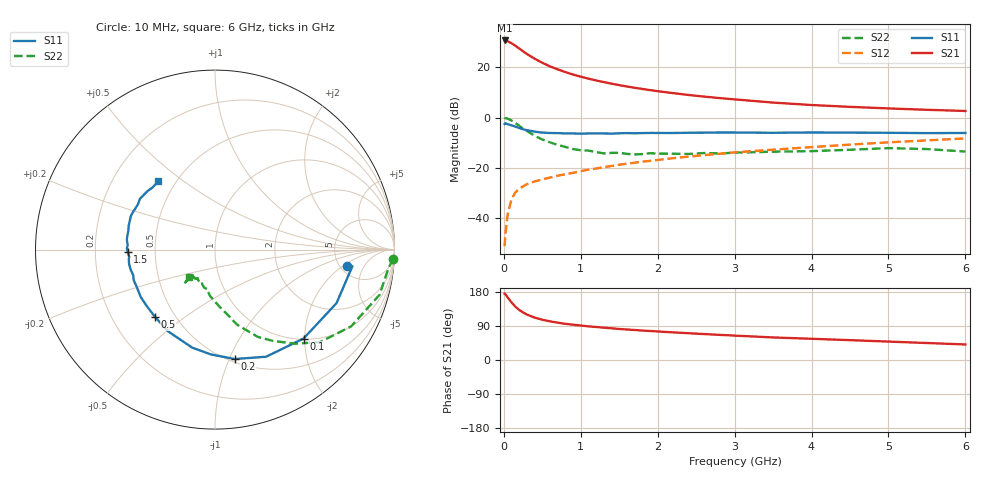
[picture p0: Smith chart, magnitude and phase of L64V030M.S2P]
!  INFINEON TECHNOLOGIES Small Signal Semiconductors
! BFR380L3 , Si-NPN RF-Transistor in TSLP-3-1
!  Vce=4 V,  Ic=30 mA
! Common Emitter S-Parameters:  07. March 2005
#  GHz  S  MA  R  50
! f  S11  S21  S12  S22
! GHz  Mag  Ang  Mag  Ang  Mag  Ang  Mag  Ang
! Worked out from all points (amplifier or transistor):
!   36 points, 10 MHz to 6 GHz, reference 50 ohm
!   highest |S21| = 30.6 dB at 10 MHz (marker M1)
!   |S21| within 3 dB of that: start of sweep to 190.8 MHz
!   unconditionally stable (mu >= 1): 1.951 GHz to 4.788 GHz
!   at 250 MHz: K = 0.37, MSG = 26.8 dB, |S12| = -27.3 dB
!   at 1.4 GHz: K = 0.95, MSG = 16.3 dB, |S12| = -19.2 dB
!   at 6 GHz: K = 0.97, MSG = 5.4 dB, |S12| = -8.3 dB
!   S11 on the Smith chart (normalised r, x): 10 MHz: 5.78, -2.41; 100 MHz: 1.02, -1.97; 200 MHz: 0.53, -1.05; 500 MHz: 0.39, -0.39; 1.5 GHz: 0.35, -0.01; 6 GHz: 0.40, +0.40
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0.01  0.744 -7.2  33.86 175.0  0.0028 80.1  0.9932 -3.0
0.02  0.7712 -6.9  33.57 174.0  0.0048 90.3  0.9716 -6.3
0.05  0.7398 -23.8  32.64 165.0  0.012 82.0  0.9506 -15.4
0.1  0.6993 -45.1  29.79 151.9  0.024 70.2  0.8709 -29.4
0.15  0.6613 -64.5  26.63 140.7  0.0326 63.2  0.7794 -41.4
0.2  0.6196 -79.7  23.41 132.1  0.0388 59.0  0.6879 -49.7
0.25  0.5843 -92.3  20.67 125.5  0.0431 55.5  0.6015 -57.7
0.3  0.5607 -103.1  18.25 119.9  0.0475 53.5  0.5425 -63.8
0.4  0.5252 -119.8  14.72 111.9  0.0539 52.5  0.4355 -73.7
0.5  0.5025 -131.7  12.21 106.3  0.0593 52.7  0.3668 -79.3
0.6  0.4932 -140.8  10.36 101.9  0.0644 53.6  0.3218 -85.1
0.7  0.4909 -147.4  9.028 98.5  0.07 54.9  0.2863 -90.6
0.9  0.4839 -159.6  7.127 93.1  0.0799 57.1  0.2367 -99.6
1.1  0.4829 -166.6  5.911 88.8  0.0924 58.9  0.2209 -105.5
1.5  0.4867 -178.3  4.399 81.9  0.1155 61.4  0.1994 -115.8
1.8  0.4915 174.9  3.693 77.7  0.133 62.5  0.1882 -121.4
2.2  0.4939 168.0  3.049 72.9  0.1561 63.2  0.1915 -125.2
2.8  0.5047 158.5  2.436 66.4  0.1907 63.8  0.1938 -132.3
3.5  0.4979 149.5  1.98 59.5  0.2304 62.3  0.2102 -132.1
4.5  0.5011 143.3  1.629 52.4  0.2902 61.3  0.2293 -132.2
5.5  0.4907 135.2  1.424 44.8  0.3522 57.9  0.2368 -132.1
6  0.494 129.8  1.349 41.0  0.3848 55.9  0.2111 -133.6
